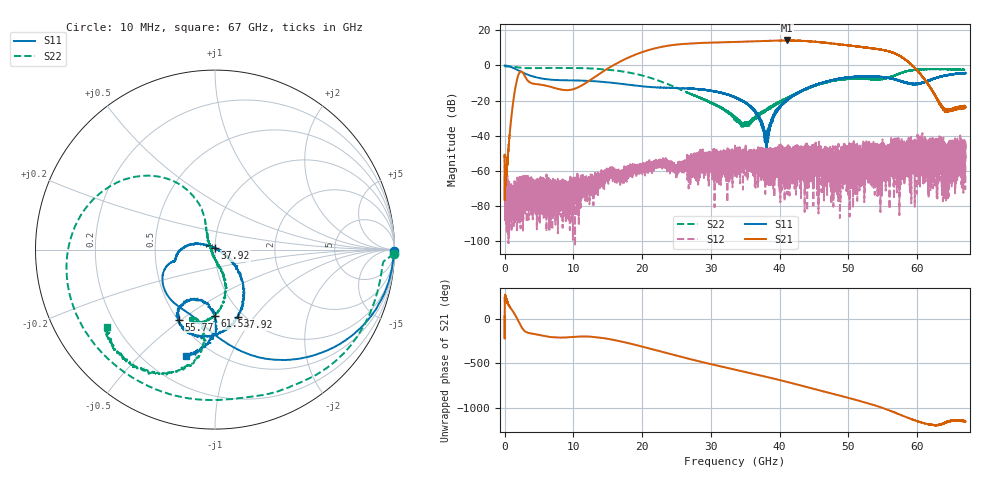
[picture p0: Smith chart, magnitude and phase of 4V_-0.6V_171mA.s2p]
! MARKI MICROWAVE INC.
! Date:  10/21/2020
! Model Number:  AMM-7210CH
! Description:  2-port Small Signal S-parameter data for AMM-7210CH
! Frequency Range:  10 MHz to 67 GHz
! Port Configuration:  PORT 1: Input
!  PORT 2: Output
! Bias Condition: Vd = +4.0V, Vg = -0.6V
! AMM-7210CH s2p files are only valid for small signal conditions (below -10 dBm input power)
# Hz S  dB  R 50
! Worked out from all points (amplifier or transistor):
!   20001 points, 10 MHz to 67 GHz, reference 50 ohm
!   highest |S21| = 14.3 dB at 41.02 GHz (marker M1)
!   |S21| within 3 dB of that: 23.78 GHz to 50.31 GHz (26.53 GHz wide, 71.6 % of centre)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
!   unconditionally stable (mu >= 1): 13.34 MHz to 16.72 MHz; 23.36 MHz to end of sweep
!   at 11.17 GHz: K = 1178.24, MAG = -5.5 dB, |S12| = -67.9 dB
!   at 33.51 GHz: K = 23.53, MAG = 13.5 dB, |S12| = -47.0 dB
!   at 67 GHz: K = 977.87, MAG = -18.2 dB, |S12| = -53.2 dB
!   S11 on the Smith chart (normalised r, x): 10 MHz: open; 37.92 GHz: 1.00, +0.02; 47.92 GHz: 0.93, -0.83; 55.77 GHz: 0.51, -0.49; 61.53 GHz: 0.76, -0.65; 67 GHz: 0.39, -0.69
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1e7  0.00 -0.5  -52.15 25.6  -51.00 -166.4  -0.02 -1.5
2.254165e9  -3.29 -63.1  -3.66 -62.7  -70.83 8.3  -1.22 -62.4
1.117723e10  -8.61 -132.9  -11.49 161.6  -69.02 -173.9  -1.51 -168.7
1.701876e10  -10.48 -159.1  2.63 104.5  -66.00 127.4  -3.34 148.5
1.991943e10  -11.83 -163.7  7.49 50.6  -59.15 113.4  -5.62 128.7
2.234112e10  -12.58 -164.1  10.20 1.6  -55.32 116.3  -8.59 115.5
2.458863e10  -12.88 -166.1  11.70 -44.5  -57.24 79.9  -12.03 108.5
2.753954e10  -13.27 -171.7  12.66 -102.0  -51.31 58.9  -17.07 111.1
3.070817e10  -14.93 177.0  13.10 -159.7  -60.33 77.9  -22.46 123.3
3.3505e10  -18.09 165.9  13.42 151.4  -47.02 51.5  -29.62 150.6
3.791629e10  -40.08 88.5  13.98 73.4  -51.28 -4.4  -25.77 -85.1
4.102463e10  -19.76 -33.5  14.27 15.2  -53.38 -100.2  -18.67 -74.8
4.271278e10  -15.45 -41.9  14.18 -18.3  -55.09 58.0  -15.46 -71.5
4.467223e10  -11.94 -52.1  13.74 -57.8  -52.42 -172.3  -12.17 -76.2
4.79246e10  -8.07 -71.4  12.41 -123.0  -53.81 147.7  -8.60 -91.5
5.128415e10  -6.31 -92.7  10.86 169.0  -77.32 58.5  -7.55 -106.8
5.376613e10  -6.26 -107.1  9.59 113.9  -56.16 -108.4  -7.95 -108.1
5.576913e10  -7.16 -117.3  8.08 60.8  -49.37 132.2  -6.94 -98.5
5.583612e10  -7.10 -117.3  8.09 59.0  -48.01 -154.9  -6.91 -98.5
5.854586e10  -9.97 -117.3  2.50 -23.9  -50.97 -155.0  -3.24 -105.1
6.153362e10  -8.62 -90.4  -10.32 -97.5  -48.73 134.3  -2.05 -123.7
6.7e10  -4.50 -105.4  -23.71 -67.2  -53.18 -109.4  -2.47 -144.5
